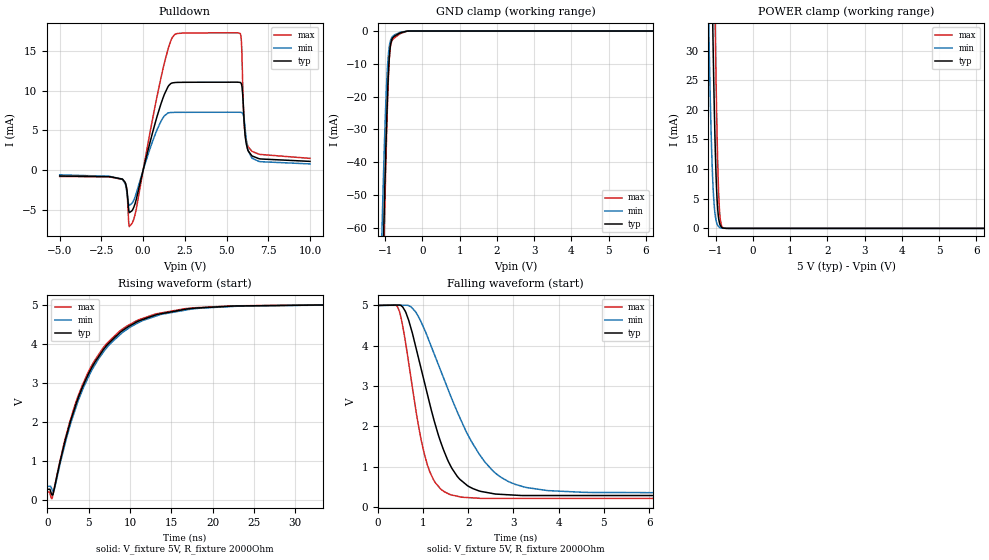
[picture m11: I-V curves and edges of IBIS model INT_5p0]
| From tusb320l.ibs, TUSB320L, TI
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|   Model
[Model]   INT_5p0
Model_type   Open_drain
Polarity   Non-Inverting
Vmeas = 2.5
Vref = 5
Cref = 1pF
Rref = 2000
|   typ   min   max
C_comp   0.595pF   0.579pF   0.649pF
[Voltage Range]   5   4.999   5.001
[Temperature Range]   27   105   -40
[Pullup Reference]   5   4.999   5.001
[Pulldown Reference]   -0   0   0
[Power Clamp Reference]   5   4.999   5.001
[GND Clamp Reference]   0   0   0
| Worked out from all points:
|   slope of the pulldown table from 0 to 0.75 V, typ, clamps not added: 122 ohm
|   GND clamp passes 1 mA (typ) near -0.67 V on its own axis
|   POWER clamp passes 1 mA (typ) near -0.90 V on its own axis
|   falling waveform, V_fixture 5V, R_fixture 2000Ohm: 20-80 % time 704ps typ, 1.11ns min, 447ps max; typ from 5 V to 0.274 V
|   rising waveform, V_fixture 5V, R_fixture 2000Ohm: 20-80 % time 5.81ns typ, 5.98ns min, 5.62ns max; typ from 0.274 V to 5 V
[Pulldown]
|   Voltage   I(typ)   I(min)   I(max)
-5V       -754uA     -602.7uA   -806.5uA
-1.25V    -1.132mA   -1.167mA   -1.173mA
-995mV    -2.219mA   -2.549mA   -2.335mA
-830mV    -5.386mA   -4.466mA   -7.144mA
-665mV    -5.13mA    -4.181mA   -6.733mA
1.27V     9.563mA    6.848mA    13.52mA
2.11V     11.08mA    7.296mA    17.27mA
5.815V    11.07mA    7.301mA    17.25mA
5.905V    10.73mA    7.265mA    15.4mA
6.055V    5.93mA     6.343mA    5.798mA
6.295V    2.424mA    2.417mA    2.943mA
10V       1.097mA    776.8uA    1.476mA
[GND Clamp]
|   Voltage   I(typ)   I(min)   I(max)
-5V       -2.346A    -2.244A    -2.423A
-1.1V     -89.8mA    -66.34mA   -99.93mA
-1.085V   -82.31mA   -59.75mA   -91.9mA
-1.04V    -60.58mA   -41.19mA   -68.42mA
-1.025V   -53.66mA   -35.51mA   -60.84mA
-965mV    -28.54mA   -16.63mA   -32.72mA
-920mV    -14.17mA   -7.851mA   -15.86mA
-890mV    -7.909mA   -4.652mA   -8.438mA
-860mV    -4.412mA   -2.944mA   -4.657mA
-830mV    -2.804mA   -2.074mA   -3.213mA
-620mV    -698.9uA   -494.3uA   -996.6uA
10V       0A         0A         0A
[POWER Clamp]
|   Voltage   I(typ)   I(min)   I(max)
-5V       2.317A     2.221A     2.385A
-1.19V    81.55mA    34.73mA    119mA
-1.13V    53.92mA    17.14mA    87.53mA
-1.085V   35.47mA    8.494mA    65.05mA
-1.025V   15.94mA    2.679mA    37.58mA
-1.01V    12.3mA     1.953mA    31.4mA
-980mV    6.741mA    1.018mA    20.31mA
-935mV    2.275mA    371.9uA    8.066mA
-905mV    1.016mA    188.3uA    3.498mA
-875mV    439.3uA    95.01uA    1.311mA
-710mV    3.815uA    2.159uA    3.074uA
10V       0A         0A         0A
[Ramp]
R_load = 2000
|   typ   min   max
dV/dt_r   2.83589/5.7751e-09   2.78968/5.94249e-09   2.87781/5.6113e-09
dV/dt_f   2.83589/7.00753e-10   2.78968/1.10843e-09   2.87781/4.45654e-10
[Falling Waveform]
V_fixture = 5V
V_fixture_min = 4.999V
V_fixture_max = 5.001V
R_fixture = 2000Ohm
C_fixture = 0F
|   Time   V(typ)   V(min)   V(max)
0s        5V         4.999V     5.001V
471.4ps   5.009V     5.004V     4.874V
683ps     4.631V     4.996V     3.578V
948.6ps   3.474V     4.613V     1.725V
1.23ns    2.207V     3.845V     679.1mV
1.637ns   960.3mV    2.682V     295.5mV
2.292ns   383.1mV    1.233V     211.6mV
3.044ns   291.7mV    558.7mV    211.6mV
4.689ns   283.3mV    359.8mV    211.5mV
200ns     273.5mV    349.5mV    204.6mV
[Rising Waveform]
V_fixture = 5V
V_fixture_min = 4.999V
V_fixture_max = 5.001V
R_fixture = 2000Ohm
C_fixture = 0F
|   Time   V(typ)   V(min)   V(max)
0s        273.5mV    349.5mV    204.6mV
586ps     129.4mV    266.8mV    37.74mV
819ps     257.7mV    240.9mV    264.4mV
2.078ns   1.444V     1.373V     1.488V
3.571ns   2.512V     2.435V     2.568V
4.943ns   3.212V     3.135V     3.27V
6.687ns   3.824V     3.759V     3.878V
11.22ns   4.603V     4.568V     4.632V
16.65ns   4.888V     4.865V     4.904V
200ns     5V         4.999V     5.001V
